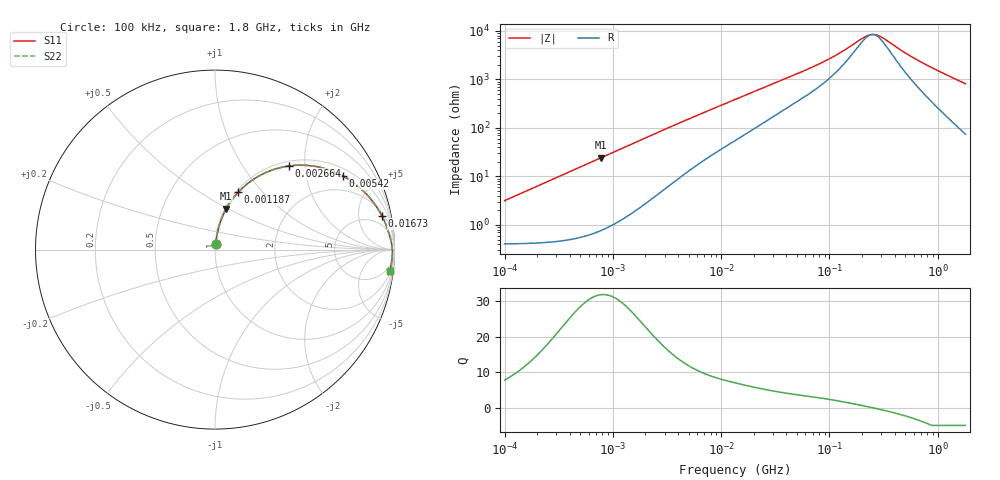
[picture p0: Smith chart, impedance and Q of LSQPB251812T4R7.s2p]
! LSQPB251812T4R7  S-PARAMETER MODEL  ( General Type )
! Model Generated by TAIYO YUDEN Corporation (http://www.ty-top.com)
! Version 3.0
! TAIYO YUDEN Control No. 110926NF18SB-HKC
! Copyright(c) 2007 TAIYO YUDEN CO.,LTD. All Rights Reserved.
! Product Description (link to TY-COMPAS)
! https://ds.yuden.co.jp/TYCOMPAS/or/detail?pn=LSQPB251812T4R7M&u=M
! Products Name : Inductors
! Characteristics :
!  Inductance : 4.7 uH , SRF(min) : 60 MHz , DC Resistance(max) : 0.52 Ohm
!  Rated Current : Saturation :700 mA , Temp Rise : 470 mA (40 degC)
!  Case Size : 2.5 x 1.8 / 0.098 x 0.071 [mm/inch] , Thickness : 1.2 / 0.048 [mm/inch]
!  (Conditions: Temperature = 25 degC , DC Bias Current/Voltage = 0A / 0V)
! External Node Assignments :
!  1  o---GGG---o  2
! GND o---------o GND
! Frequency Range : 0.1MHz  -  1800MHz  [ 402 STEP ]
# MHz S RI R 50
! Freq[MHz].  S11 Real  S11 Imag  S21 Real  S21 Imag  S12 Real  S12 Imag  S22 Real  S22 Imag
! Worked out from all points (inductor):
!   401 points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, 100 kHz to 1.8 GHz, reference 50 ohm
!   read as one part in series: L = 5 uH near 105 kHz
!   highest Q = 31.8 at 782.7 kHz (marker M1), where L = 4.99 uH
!   self-resonance near 248.8 MHz
!   S11 on the Smith chart (normalised r, x): 100 kHz: 1.01, +0.06; 1.187 MHz: 1.02, +0.74; 2.664 MHz: 1.09, +1.66; 5.42 MHz: 1.29, +3.29; 16.73 MHz: 2.48, +9.36; 1.8 GHz: 2, -16
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0.1  0.00502 0.0311  0.995 -0.0311  0.995 -0.0311  0.00502 0.0311
0.247521  0.0103 0.0766  0.9897 -0.0766  0.9897 -0.0766  0.0103 0.0766
0.516129  0.0308 0.1562  0.9692 -0.1562  0.9692 -0.1562  0.0308 0.1562
0.782721  0.0633 0.2283  0.9367 -0.2283  0.9367 -0.2283  0.0633 0.2283
1.187015  0.1298 0.3197  0.8702 -0.3197  0.8702 -0.3197  0.1298 0.3197
1.756577  0.2408 0.4078  0.7592 -0.4078  0.7592 -0.4078  0.2408 0.4078
2.66389  0.412 0.466  0.588 -0.466  0.588 -0.466  0.412 0.466
3.753625  0.5684 0.4619  0.4316 -0.4619  0.4316 -0.4619  0.5684 0.4619
5.420303  0.7143 0.4093  0.2857 -0.4093  0.2857 -0.4093  0.7143 0.4093
8.220015  0.8304 0.3228  0.1696 -0.3228  0.1696 -0.3228  0.8304 0.3228
13.41641  0.9089 0.2249  0.0911 -0.2249  0.0911 -0.2249  0.9089 0.2249
16.72553  0.9301 0.1877  0.0699 -0.1877  0.0699 -0.1877  0.9301 0.1877
31.62078  0.9636 0.1077  0.0364 -0.1077  0.0364 -0.1077  0.9636 0.1077
69.24595  0.9803 0.0511  0.0197 -0.0511  0.0197 -0.0511  0.9803 0.0511
115.8234  0.9854 0.0272  0.0146 -0.0272  0.0146 -0.0272  0.9854 0.0272
198.5346  0.9879 0.00754  0.0121 -0.00754  0.0121 -0.00754  0.9879 0.00754
229.9669  0.9882 0.00262  0.0118 -0.00262  0.0118 -0.00262  0.9882 0.00262
253.6402  0.9883 -0.000642  0.0117 0.000642  0.0117 0.000642  0.9883 -0.000642
279.7504  0.9884 -0.00392  0.0116 0.00392  0.0116 0.00392  0.9884 -0.00392
357.3983  0.9885 -0.0124  0.0115 0.0124  0.0115 0.0124  0.9885 -0.0124
692.4421  0.9872 -0.0406  0.0128 0.0406  0.0128 0.0406  0.9872 -0.0406
1800  0.9748 -0.1176  0.0252 0.1176  0.0252 0.1176  0.9748 -0.1176
